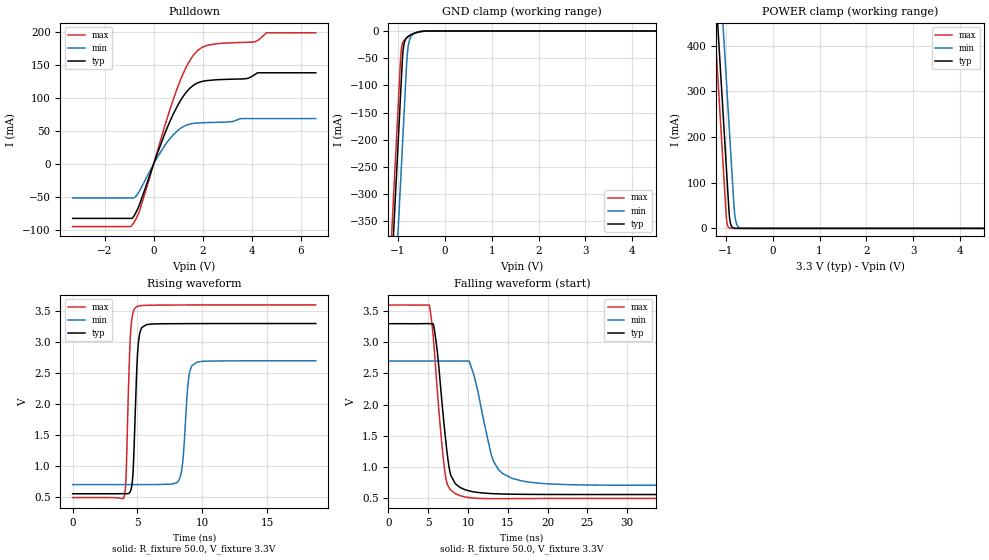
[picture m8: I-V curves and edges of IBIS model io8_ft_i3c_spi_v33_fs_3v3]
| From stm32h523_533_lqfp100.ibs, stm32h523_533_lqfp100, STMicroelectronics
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[Model]   io8_ft_i3c_spi_v33_fs_3v3
Model_type I/O_open_drain
Polarity   Non-Inverting
Enable   Active-Low
| CAP_THRESHOLD on pad IOFT is "UDTCAPC" :
| Rising=20.0% of vddiom   Falling=80.0% of vddiom
| C_comp min and max val. don't necessarily correlate with the min and max pvt
| but are the smallest and greatest pad capacitance found.
| var   typ   min   max
C_comp   3.95302pF  3.95027pF  4.00767pF
|C_comp_pulldown   3.95302pF  3.95027pF  4.00767pF
Vinl = 1.35V
Vinh = 1.8V
Vmeas = 1.65V   | Reference voltage for timing measurements
Cref  = 50.0pF   | Timing specification test load capacitance value
Rref  = 1.0MOhm   | Timing specification test load resistance value
Vref  = 1.815V   | Timing specification test load voltage
[Model Spec]
| TIME_THRESHOLD on pin ZII2CV11 is "CMOS" :
| Rising=40.0% of vdd   Falling=60.0% of vdd
Vinl 1.28680V 1.06380V 1.39380V
Vinh 1.76920V 1.48820V 1.89120V
| variable   typ   min   max
[Temperature Range] 25.0 125.0 -40.0
| variable   typ   min   max
[Voltage Range] 3.3V 2.7V 3.6V
| variable   typ   min   max
[POWER Clamp Reference] 3.3V 2.7V 3.6V
| variable   typ   min   max
[GND Clamp Reference] 0V 0V 0V
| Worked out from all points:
|   slope of the pulldown table from 0 to 0.495 V, typ, clamps not added: 10 ohm
|   GND clamp passes 1 mA (typ) near -0.52 V on its own axis
|   POWER clamp passes 1 mA (typ) near -0.84 V on its own axis
|   rising waveform, R_fixture 50.0, V_fixture 3.3V: 20-80 % time 285ps typ, 380ps min, 266ps max; typ from 0.556 V to 3.3 V
|   falling waveform, R_fixture 50.0, V_fixture 3.3V: 20-80 % time 1.27ns typ, 2.09ns min, 1.21ns max; typ from 3.3 V to 0.556 V
[POWER Clamp]
-3.3V     4.068A     4.259A     3.957A
-1.25V    582.8mA    774.2mA    471.5mA
-1.21V    514.8mA    706.2mA    403.5mA
-1.13V    378.8mA    570.2mA    267.5mA
-1.04V    225.8mA    417.2mA    114.5mA
-980mV    123.8mA    315.2mA    17.95mA
-920mV    26.3mA     213.2mA    906uA
-880mV    5.543mA    145.2mA    123.7uA
-810mV    363.5uA    33.6mA     3.798uA
-770mV    76.62uA    10.47mA    519.4nA
-690mV    3.409uA    1.017mA    10.47nA
6.6V      0A         0A         0A
[GND Clamp]
-3.3V     -4.13A     -4.291A    -4.063A
-1.25V    -644.7mA   -806.4mA   -578.1mA
-940mV    -117.7mA   -279.4mA   -51.06mA
-920mV    -83.75mA   -245.4mA   -31.43mA
-900mV    -50.5mA    -211.4mA   -23.14mA
-880mV    -31.27mA   -177.4mA   -19.1mA
-850mV    -18.68mA   -126.4mA   -15.73mA
-800mV    -11.46mA   -46.4mA    -12.03mA
-760mV    -8.752mA   -20.02mA   -9.606mA
-680mV    -5.122mA   -6.673mA   -5.579mA
-300mV    -5.379uA   -47.63uA   -852.7nA
6.6V      10.49nA    1.843uA    393.6pA
| variable   typ   min   max
[Pullup Reference] 3.3V 2.7V 3.6V
| variable   typ   min   max
[Pulldown Reference] 0V 0V 0V
[Pulldown]
-3.3V     -82.42mA   -51.49mA   -94.82mA
-850mV    -81.27mA   -51.49mA   -91.26mA
-580mV    -62.01mA   -41.36mA   -71.41mA
120mV     12.61mA    7.999mA    15.37mA
800mV     75.3mA     43.94mA    97.52mA
1.33V     108.3mA    58.37mA    146.5mA
1.84V     123.1mA    61.83mA    172.7mA
2.51V     126.9mA    62.7mA     181.3mA
3.78V     128.8mA    68.32mA    183.7mA
4.12V     134.9mA    68.32mA    184.6mA
4.59V     137.6mA    68.32mA    198mA
6.6V      137.6mA    68.32mA    198mA
[Ramp]
dV/dt_r 1.64659V/282.77362ps 1.19782V/377.48552ps 1.86382V/262.637ps
dV/dt_f 1.64666V/1.26935ns 1.19801V/2.06866ns 1.86387V/1.20921ns
R_load = 50.0
| Removed startup time: 0s 0s 0s  .
| Removed end time: 18.75ns.
[Rising Waveform]
R_fixture   = 50.0
V_fixture   = 3.3V
V_fixture_min = 2.7V
V_fixture_max = 3.6V
0s        555.6mV    703.3mV    493.6mV
3.95ns    557.7mV    703.3mV    494mV
4.1ns     556.5mV    703.3mV    723.3mV
4.6ns     738.2mV    703.3mV    3.416V
4.9ns     2.288V     703.3mV    3.564V
5.35ns    3.238V     703.3mV    3.59V
8.2ns     3.298V     776.3mV    3.599V
8.95ns    3.298V     2.419V     3.599V
9.6ns     3.299V     2.679V     3.599V
18.75ns   3.3V       2.7V       3.6V
| Removed startup time: 0s 0s 0s  .
| Removed end time: 58.7ns.
[Falling Waveform]
R_fixture   = 50.0
V_fixture   = 3.3V
V_fixture_min = 2.7V
V_fixture_max = 3.6V
0s        3.3V       2.7V       3.6V
5.15ns    3.301V     2.7V       3.593V
6ns       3.008V     2.7V       2.48V
7.2ns     1.43V      2.7V       833.7mV
7.85ns    862.9mV    2.7V       626.4mV
8.95ns    673.6mV    2.701V     539.5mV
10.2ns    612mV      2.683V     505.7mV
13.2ns    569.2mV    1.091V     488.7mV
15.6ns    560.9mV    813mV      489.5mV
58.7ns    555.6mV    703.3mV    493.6mV
